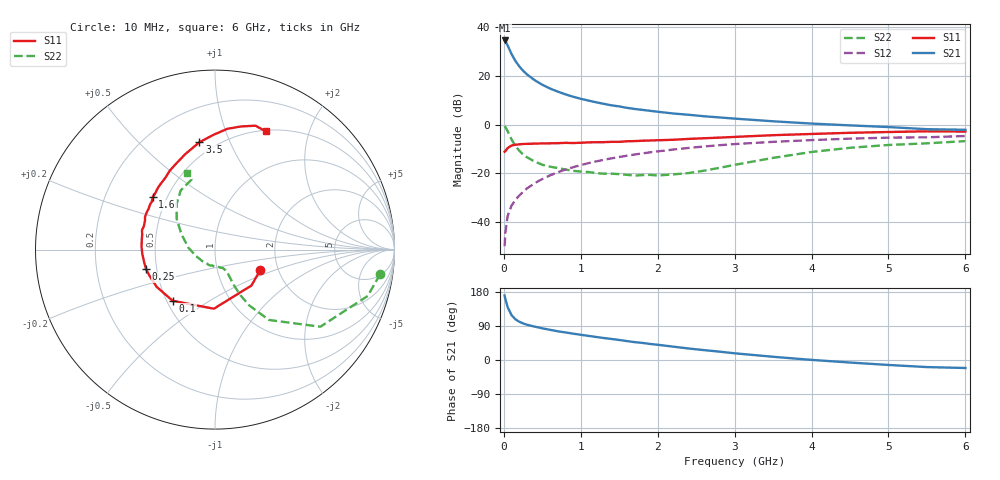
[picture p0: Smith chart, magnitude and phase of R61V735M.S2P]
! SIEMENS Small Signal Semiconductors
! BFR193
! Si NPN RF Bipolar Junction Transistor in SOT23
! VCE = 1.75 V  IC = 35 mA
! Common Emitter S-Parameters:  May  1996
# GHz  S  MA  R  50
!  f  S11  S21  S12  S22
! GHz  MAG  ANG  MAG  ANG  MAG  ANG  MAG  ANG
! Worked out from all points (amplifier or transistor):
!   36 points, 10 MHz to 6 GHz, reference 50 ohm
!   highest |S21| = 34.5 dB at 10 MHz (marker M1)
!   |S21| within 3 dB of that: start of sweep to 63.26 MHz
!   unconditionally stable (mu >= 1): 416.8 MHz to 1.957 GHz
!   at 250 MHz: K = 0.93, MSG = 24.8 dB, |S12| = -27.6 dB
!   at 1.4 GHz: K = 1.02, MAG = 9.9 dB, |S12| = -13.9 dB
!   at 6 GHz: K = 0.96, MSG = 1.3 dB, |S12| = -4.7 dB
!   S11 on the Smith chart (normalised r, x): 10 MHz: 1.62, -0.40; 100 MHz: 0.54, -0.35; 250 MHz: 0.44, -0.11; 1.6 GHz: 0.42, +0.31; 3.5 GHz: 0.41, +0.78; 6 GHz: 0.51, +1.39
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0.01  0.2769 -24.1  52.96 170.2  0.0032 83.9  0.93 -8.5
0.02  0.2852 -44.6  50.91 160.9  0.0061 81.6  0.8891 -16.9
0.05  0.3295 -91.1  41.71 138.9  0.0135 69.3  0.7275 -36.2
0.1  0.3701 -129.6  27.91 118.5  0.0217 66.0  0.4943 -52.5
0.15  0.3856 -147.4  20.17 107.5  0.0284 67.0  0.3646 -58.5
0.2  0.3921 -157.4  15.66 101.0  0.0349 69.6  0.2911 -60.9
0.25  0.3994 -164.1  12.67 96.6  0.0416 70.5  0.2434 -61.7
0.3  0.4009 -169.7  10.69 93.1  0.0487 71.5  0.2137 -62.0
0.4  0.4058 -176.8  8.133 88.1  0.0625 72.5  0.1742 -61.8
0.5  0.4094 177.8  6.535 83.6  0.0763 72.8  0.1497 -61.6
0.6  0.4115 172.6  5.475 79.7  0.0905 72.1  0.1366 -62.2
0.7  0.4143 168.3  4.735 75.8  0.1047 71.4  0.1282 -63.2
0.9  0.4175 161.4  3.713 69.6  0.1332 69.3  0.112 -66.4
1.1  0.4303 154.9  3.094 63.6  0.1614 66.9  0.1062 -72.8
1.3  0.4347 148.1  2.656 58.0  0.1892 64.1  0.098 -79.5
1.6  0.4534 139.9  2.199 49.9  0.2292 59.8  0.093 -94.7
2.2  0.4864 124.7  1.685 35.3  0.3065 50.8  0.0948 -132.9
3  0.5568 107.4  1.322 17.7  0.3973 37.9  0.1489 175.7
3.5  0.6044 98.3  1.165 8.5  0.4413 29.9  0.2069 155.0
4.5  0.6764 84.2  0.96 -6.7  0.5132 15.7  0.3331 129.9
5.5  0.7263 71.9  0.802 -18.7  0.5468 1.8  0.4115 108.6
6  0.7168 66.7  0.78 -21.1  0.5811 -2.3  0.4568 110.2
